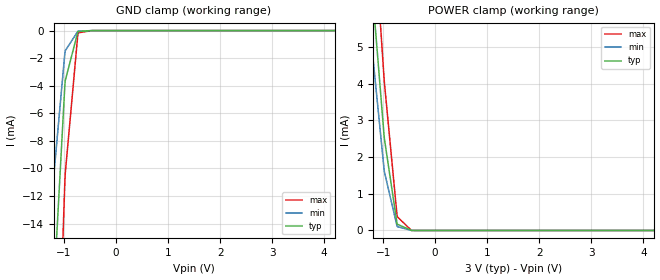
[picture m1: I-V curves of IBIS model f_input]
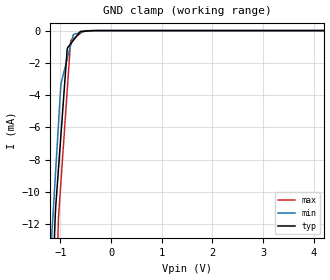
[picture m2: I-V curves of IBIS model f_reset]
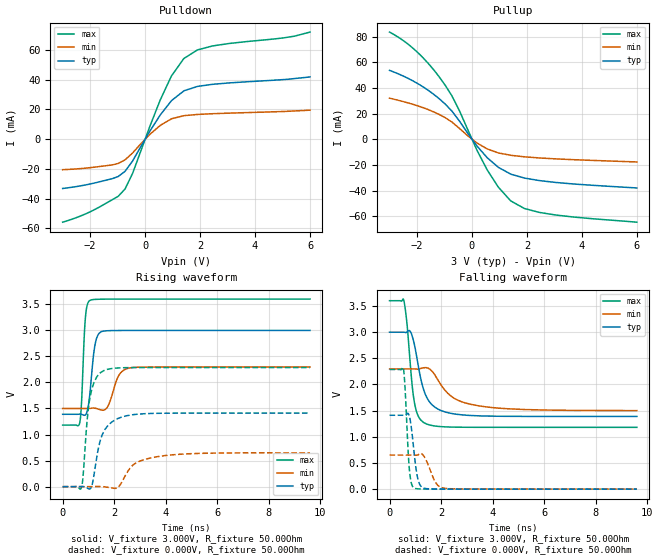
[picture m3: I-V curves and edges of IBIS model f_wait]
[IBIS Ver]   3.2
[File Name]   p33_30v_512m_65nm_b.ibs
[File Rev]   1.01
[Date]   9/9/2009
[Source]   From silicon level SPICE model at Numonyx B.V.
[Notes]   The following information corresponds to the 65nm P33
   512Mb chip with EzBGA package.
[Disclaimer]   This information is for modeling purposes only and is not
   guaranteed.Numonyx B.V. is not responsible for any problem
   this model may cause to customers.
[Copyright]   Copyright 2009, Numonyx B.V., All Rights Reserved.
[Component]   P33_30V_512M_EZBGA
[Manufacturer]  Numonyx B.V.
[Package]
|   typ   min   max
R_pkg   0.40Ohm   0.13Ohm   0.67Ohm
L_pkg   8.65nH   2.98nH   14.32nH
C_pkg   1.17pF   0.26pF   2.08pF
[PIN]   signal_name   model_name   R_pin   L_pin   C_pin
A1   A1   f_input   0.47   9.18nH   1.16pF
A2   A6   f_input   0.26   5.46nH   0.58pF
A3   A8   f_input   0.13   2.98nH   0.29pF
A4   VPP   POWER
A5   A13   f_input   0.28   5.89nH   0.66pF
A6   VCC   POWER
A7   A18   f_input   0.28   6.05nH   0.69pF
A8   A22   f_input   0.34   6.88nH   0.80pF
B1   A2   f_input   0.20   4.18nH   0.37pF
B2   VSS   GND
B3   A9   f_input   0.27   5.80nH   0.65pF
B4   CE#   f_input   0.45   8.83nH   1.10pF
B5   A14   f_input   0.28   5.89nH   0.65pF
B6   A25   f_input   0.52   9.67nH   1.22pF
B7   A19   f_input   0.45   8.60nH   1.16pF
B8   NC   NC
C1   A3   f_input   0.24   4.84nH   0.46pF
C2   A7   f_input   0.25   5.33nH   0.56pF
C3   A10   f_input   0.39   8.42nH   1.09pF
C4   A12   f_input   0.49   9.97nH   1.33pF
C5   A15   f_input   0.41   7.86nH   0.95pF
C6   WP#   f_input   0.26   5.46nH   0.59pF
C7   A20   f_input   0.47   8.74nH   1.15pF
C8   A21   f_input   0.28   5.82nH   0.63pF
D1   A4   f_input   0.29   6.08nH   0.68pF
D2   A5   f_input   0.25   5.17nH   0.53pF
D3   A11   f_input   0.55   9.98nH   1.26pF
D4   RST#   f_reset   0.35   6.81nH   0.77pF
D5   VCCQ   POWER
D6   VCCQ   POWER
D7   A16   f_input   0.30   5.86nH   0.70pF
D8   A17   f_input   0.33   6.41nH   0.70pF
E1   DQ8   f_inout   0.36   7.05nH   0.81pF
E2   DQ1   f_inout   0.33   6.32nH   0.69pF
E3   DQ9   f_inout   0.25   5.03nH   0.56pF
E4   DQ3   f_inout   0.25   5.00nH   0.55pF
E5   DQ4   f_inout   0.28   5.52nH   0.56pF
E6   CLK   f_input   0.27   5.42nH   0.55pF
E7   DQ15   f_inout   0.27   5.27nH   0.60pF
E8   NC   NC
F1   NC   NC
F2   DQ0   f_inout   0.24   4.94nH   0.57pF
F3   DQ10   f_inout   0.25   4.93nH   0.53pF
F4   DQ11   f_inout   0.20   4.19nH   0.43pF
F5   DQ12   f_inout   0.23   4.71nH   0.44pF
F6   ADV#   f_input   0.21   4.27nH   0.43pF
F7   WAIT   f_wait   0.23   4.62nH   0.51pF
F8   OE#   f_input   0.46   9.68nH   1.29pF
G1   A23   f_input   0.60   13.06nH   1.64pF
G2   NC   NC
G3   DQ2   f_inout   0.26   5.27nH   0.62pF
G4   VCCQ   POWER
G5   DQ5   f_inout   0.23   4.73nH   0.45pF
G6   DQ6   f_inout   0.25   5.05nH   0.49pF
G7   DQ14   f_inout   0.19   3.91nH   0.40pF
G8   WE#   f_input   0.46   9.41nH   1.10pF
H1   NC   NC
H2   VSS   GND
H3   VCC   POWER
H4   VSS   GND
H5   DQ13   f_inout   0.25   5.25nH   0.54pF
H6   VSSQ   GND
H7   DQ7   f_inout   0.13   2.99nH   0.26pF
H8   A24   f_input   0.67   14.32nH   2.08pF
| Models and submodels in the file (4): f_input (Input), f_reset (Input), f_wait (Output), f_inout (I/O)
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[Model]   f_input
Model_type   Input
Vinl = 0.400V
Vinh = 2.600V
|   typ   min   max
C_comp   4.280pF   2.270pF   4.770pF
[Voltage Range]   3.000V   2.300V   3.600V
[Temperature Range]   25.0   85.0   -40.0
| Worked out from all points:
|   GND clamp passes 1 mA (typ) near -0.79 V on its own axis
|   POWER clamp passes 1 mA (typ) near -0.82 V on its own axis
[GND Clamp]
|   Voltage   I(typ)   I(min)   I(max)
-3V       -214.2mA   -171.1mA   -282mA
-1.398V   -38.01mA   -24.9mA    -60.4mA
-1.209V   -20.02mA   -11.33mA   -36.27mA
-1.2V     -19.19mA   -10.72mA   -35.15mA
-984mV    -4.085mA   -1.721mA   -11.16mA
-975mV    -3.631mA   -1.46mA    -10.38mA
-732mV    -88.55uA   -49.57uA   -226.8uA
-723mV    -64.96uA   -39.8uA    -159.9uA
-453mV    -377.4nA   -554.6nA   -216.8nA
6V        0A         0A         0A
[POWER Clamp]
|   Voltage   I(typ)   I(min)   I(max)
-3V       44.58mA    39.22mA    51.64mA
-1.299V   8.339mA    6.46mA     11.02mA
-1.209V   6.572mA    4.919mA    8.979mA
-1.2V     6.398mA    4.769mA    8.776mA
-984mV    2.624mA    1.697mA    4.188mA
-975mV    2.493mA    1.595mA    4.017mA
-732mV    187.3uA    115.4uA    401uA
-723mV    168.4uA    103.4uA    368.4uA
-453mV    1.105uA    1.525uA    700.3nA
6V        0A         0A         0A
[Model]   f_reset
Model_type   Input
Vinl = 0.400V
Vinh = 2.600V
|   typ   min   max
C_comp   2.620pF   1.330pF   2.700pF
[Voltage Range]   3.000V   2.300V   3.600V
[Temperature Range]   25.0   85.0   -40.0
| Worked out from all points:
|   GND clamp passes 1 mA (typ) near -0.84 V on its own axis
[GND Clamp]
|   Voltage   I(typ)   I(min)   I(max)
-3V       -205.4mA   -173mA     -256.3mA
-1.209V   -20.5mA    -14.72mA   -29.6mA
-1.101V   -11.42mA   -9.082mA   -18.23mA
-1.047V   -8.959mA   -6.264mA   -12.54mA
-1.038V   -8.571mA   -5.795mA   -11.6mA
-993mV    -6.627mA   -3.447mA   -9.54mA
-867mV    -1.187mA   -1.777mA   -3.783mA
-795mV    -811.6uA   -873.4uA   -609.4uA
-741mV    -594.7uA   -238.1uA   -486.6uA
-606mV    -54.38uA   -121.6uA   -179.4uA
-318mV    -41.02nA   -2.805uA   -2.579uA
6V        0A         0A         0A
[POWER Clamp]
|   Voltage   I(typ)   I(min)   I(max)
-3V       0A         0A         0A
0V        0A         0A         0A
2.301V    0A         0A         0A
3.003V    0A         0A         0A
3.597V    0A         0A         0A
6V        0A         0A         0A
[Model]   f_wait
Model_type   Output
Vmeas = 1.500V
Cref = 30.000pF
|   typ   min   max
C_comp   4.245pF   3.750pF   4.660pF
[Voltage Range]   3.000V   2.300V   3.600V
[Temperature Range]   25.0   85.0   -40.0
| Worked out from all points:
|   slope of the pulldown table from 0 to 0.45 V, typ, clamps not added: 33.4 ohm
|   slope of the pullup table from 0 to 0.45 V, typ, clamps not added: 37.7 ohm
|   falling waveform, V_fixture 3.000V, R_fixture 50.00Ohm: 20-80 % time 491ps typ, 1.04ns min, 277ps max; typ from 3 V to 1.39 V
|   rising waveform, V_fixture 3.000V, R_fixture 50.00Ohm: 20-80 % time 200ps typ, 330ps min, 126ps max; typ from 1.39 V to 3 V
|   rising waveform, V_fixture 0.000V, R_fixture 50.00Ohm: 20-80 % time 454ps typ, 827ps min, 281ps max; typ from 0.001 V to 1.41 V
|   falling waveform, V_fixture 0.000V, R_fixture 50.00Ohm: 20-80 % time 206ps typ, 331ps min, 144ps max; typ from 1.41 V to 0.001 V
[Pulldown]
|   Voltage   I(typ)   I(min)   I(max)
-3V       -33.17mA   -20.53mA   -55.87mA
-1.749V   -29.08mA   -18.62mA   -46.54mA
-984mV    -25.16mA   -16.36mA   -38.49mA
-732mV    -21.66mA   -13.91mA   -33.56mA
-453mV    -14.6mA    -9.238mA   -22.92mA
555mV     16.41mA    9.352mA    26.57mA
960mV     25.94mA    13.72mA    42.61mA
1.41V     32.52mA    15.82mA    54.32mA
1.905V    35.51mA    16.65mA    60.11mA
2.454V    36.94mA    17.15mA    62.78mA
5.055V    40.16mA    18.66mA    68.25mA
6V        41.95mA    19.57mA    72.1mA
[Pullup]
|   Voltage   I(typ)   I(min)   I(max)
-3V       53.65mA    32.02mA    83.45mA
-2.028V   44.02mA    26.42mA    68.6mA
-1.2V     31.72mA    19.39mA    48.84mA
-723mV    21.78mA    13.32mA    33.51mA
-453mV    14.08mA    8.415mA    22.06mA
177mV     -5.082mA   -2.795mA   -8.314mA
546mV     -14.15mA   -7.403mA   -23.55mA
960mV     -21.82mA   -10.61mA   -37.28mA
1.41V     -27.11mA   -12.44mA   -47.96mA
1.905V    -30.16mA   -13.63mA   -53.85mA
2.454V    -32.15mA   -14.53mA   -56.94mA
6V        -37.9mA    -17.65mA   -64.54mA
[Ramp]
R_load = 50.00Ohm
|   typ   min   max
dV/dt_r   846.106mV/453.920ps 389.161mV/825.006ps   1.371V/280.625ps
dV/dt_f   964.716mV/490.385ps 477.104mV/1.043ns   1.450V/276.963ps
[Falling Waveform]
V_fixture = 3.000V
V_fixture_min = 2.300V
V_fixture_max = 3.600V
R_fixture = 50.00Ohm
|   Time   V(typ)   V(min)   V(max)
0s        2.997V     2.296V     3.598V
550ps     2.997V     2.296V     3.611V
670ps     2.996V     2.296V     3.196V
780ps     3.026V     2.296V     2.548V
960ps     2.772V     2.296V     1.674V
1.34ns    1.876V     2.319V     1.268V
1.89ns    1.526V     2.075V     1.199V
2.44ns    1.443V     1.758V     1.186V
3.18ns    1.406V     1.617V     1.182V
9.6ns     1.389V     1.501V     1.181V
[Rising Waveform]
V_fixture = 3.000V
V_fixture_min = 2.300V
V_fixture_max = 3.600V
R_fixture = 50.00Ohm
|   Time   V(typ)   V(min)   V(max)
0s        1.389V     1.501V     1.181V
660ps     1.392V     1.501V     1.219V
730ps     1.389V     1.501V     1.586V
880ps     1.377V     1.501V     3.221V
1.07ns    1.849V     1.503V     3.575V
1.26ns    2.731V     1.505V     3.591V
1.53ns    2.977V     1.467V     3.595V
2.19ns    2.995V     2.141V     3.597V
2.56ns    2.996V     2.273V     3.598V
9.6ns     2.997V     2.296V     3.598V
[Rising Waveform]
V_fixture = 0.000V
V_fixture_min = 0.000V
V_fixture_max = 0.000V
R_fixture = 50.00Ohm
|   Time   V(typ)   V(min)   V(max)
0s        1.433mV    2.561mV    949.3uV
730ps     4.623mV    2.562mV    -14.29mV
790ps     3.815mV    2.567mV    188.5mV
960ps     -27.51mV   2.474mV    1.322V
1.07ns    -38.49mV   1.817mV    1.731V
1.59ns    1.053V     358uV      2.225V
2.11ns    1.299V     -23.68mV   2.276V
2.74ns    1.382V     419.3mV    2.284V
3.68ns    1.407V     576.5mV    2.285V
9.6ns     1.412V     651.2mV    2.285V
[Falling Waveform]
V_fixture = 0.000V
V_fixture_min = 0.000V
V_fixture_max = 0.000V
R_fixture = 50.00Ohm
|   Time   V(typ)   V(min)   V(max)
0s        1.412V     651.2mV    2.285V
540ps     1.412V     651.2mV    2.299V
600ps     1.409V     651.2mV    1.95V
770ps     1.393V     651.2mV    382.6mV
960ps     671.7mV    651.3mV    22.54mV
1.13ns    144mV      662.8mV    6.45mV
1.39ns    14.15mV    584.2mV    2.837mV
1.81ns    3.687mV    111.7mV    1.496mV
2.16ns    2.488mV    16.8mV     1.155mV
9.6ns     1.433mV    2.561mV    949.3uV
